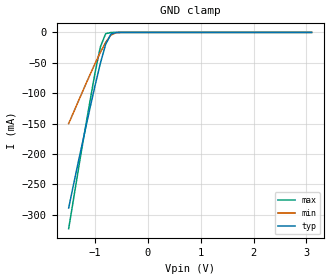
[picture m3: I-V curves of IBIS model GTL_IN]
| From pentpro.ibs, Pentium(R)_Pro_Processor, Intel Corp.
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[Model]   GTL_IN
Model_type  Input
Polarity   Inverting
Enable   Active-Low
Vinl = 0.8
Vinh = 1.2
|Variable   typ   min   max
C_comp   3.0p   2.7p   3.3p
|Variable   typ   min   max
[Voltage range] 3.1   2.845   3.255
|Variable   typ   min   max
[Temperature Range] 80   0   100
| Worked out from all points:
|   GND clamp passes 1 mA (typ) near -0.63 V on its own axis
[GND_clamp]
|Volts   typ   min   max
-1.5V     -289mA     -150mA     -323mA
-1.3V     -206mA     -110mA     -217mA
-1.2V     -166mA     -89.9mA    -165mA
-1V       -87.3mA    -51.2mA    -66.2mA
-900mV    -50.9mA    -32.9mA    -23.9mA
-800mV    -19.7mA    -16.4mA    -2.14mA
-700mV    -2.72mA    -4.27mA    -134uA
-600mV    -187uA     -406uA     -8.1uA
3.1V      0A         0A         0A
[POWER_clamp]
|Volts   typ   min   max
-600mV    0A         0A         0A
0V        0A         0A         0A
